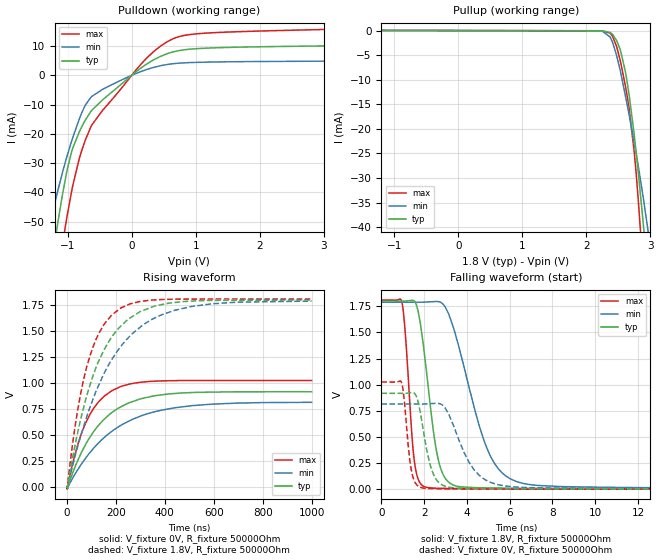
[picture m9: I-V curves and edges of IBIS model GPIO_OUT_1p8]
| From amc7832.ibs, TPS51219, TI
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|   Model
[Model]   GPIO_OUT_1p8
Model_type   Output
Polarity   Non-Inverting
Vmeas = 0.9
Vref = 1.8
Cref = 1pF
Rref = 1000000
|   typ   min   max
C_comp   1pF   1pF   1pF
[Voltage Range]   1.8   1.79   1.81
[Temperature Range]   27   125   -40
[Pullup Reference]   1.8   1.79   1.81
[Pulldown Reference]   -0   -0   -0
[Power Clamp Reference]   1.8   1.79   1.81
[GND Clamp Reference]   -0   -0   -0
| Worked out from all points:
|   slope of the pulldown table from 0 to 0.27 V, typ, clamps not added: 62.1 ohm
|   slope of the pullup table from 0 to 0.27 V, typ, clamps not added: 48 kohm
|   falling waveform, V_fixture 1.8V, R_fixture 50000Ohm: 20-80 % time 660ps typ, 1.47ns min, 358ps max; typ from 1.8 V to 0.004 V
|   rising waveform, V_fixture 0V, R_fixture 50000Ohm: 20-80 % time 163ns typ, 226ns min, 109ns max; typ from 0.002 V to 0.918 V
|   rising waveform, V_fixture 1.8V, R_fixture 50000Ohm: 20-80 % time 152ns typ, 208ns min, 104ns max; typ from 0.004 V to 1.8 V
|   falling waveform, V_fixture 0V, R_fixture 50000Ohm: 20-80 % time 532ps typ, 1.15ns min, 296ps max; typ from 0.918 V to 0.002 V
[Pulldown]
|   Voltage   I(typ)   I(min)   I(max)
-1.8V     -153.5mA   -105.7mA   -209mA
-1.309V   -73.18mA   -53.88mA   -99.6mA
-1.168V   -52.55mA   -40.82mA   -71.78mA
-1.082V   -41.03mA   -33.39mA   -58mA
-1.017V   -33.45mA   -28.23mA   -49.31mA
-919.8mV  -24.93mA   -21.36mA   -37.74mA
-784.8mV  -17.87mA   -13.12mA   -26.12mA
-622.8mV  -11.97mA   -7.251mA   -17.02mA
154.8mV   2.634mA    1.352mA    4.008mA
559.8mV   7.408mA    3.695mA    11.5mA
1.138V    9.23mA     4.469mA    14.36mA
3.595V    10.18mA    4.865mA    15.94mA
[Pullup]
|   Voltage   I(typ)   I(min)   I(max)
-1.8V     37.49uA    30.22uA    47.14uA
2.147V    -45.6uA    -47.64uA   -56.55uA
2.369V    -385.3uA   -1.286mA   -520.2uA
2.471V    -2.035mA   -5.037mA   -3.243mA
2.52V     -3.597mA   -7.642mA   -5.638mA
2.628V    -9.791mA   -14.5mA    -12.64mA
2.741V    -20.59mA   -22.4mA    -24.04mA
2.812V    -29.09mA   -27.69mA   -34.73mA
2.882V    -38.44mA   -33.47mA   -47.71mA
2.893V    -39.94mA   -34.39mA   -49.83mA
3.038V    -61.2mA    -47.6mA    -80.07mA
3.595V    -152.1mA   -106mA     -204.8mA
[Ramp]
R_load = 50000
|   typ   min   max
dV/dt_r   0.54985/1.6255e-07   0.488051/2.25521e-07   0.614753/1.08572e-07
dV/dt_f   1.07777/6.6e-10   1.06994/1.46783e-09   1.08424/3.57833e-10
[Falling Waveform]
V_fixture = 1.8V
V_fixture_min = 1.79V
V_fixture_max = 1.81V
R_fixture = 50000Ohm
C_fixture = 0F
|   Time   V(typ)   V(min)   V(max)
0s        1.8V       1.79V      1.81V
984.2ps   1.8V       1.79V      1.768V
1.466ns   1.808V     1.79V      423mV
1.73ns    1.693V     1.79V      92.9mV
2.711ns   243.4mV    1.794V     9.714mV
3.805ns   22.78mV    1.219V     6.281mV
4.99ns    14.15mV    366.8mV    5.045mV
6.018ns   11.18mV    101.9mV    4.367mV
14.03ns   4.765mV    13.88mV    3.009mV
1us       3.902mV    6.729mV    2.919mV
[Rising Waveform]
V_fixture = 0V
V_fixture_min = 0V
V_fixture_max = 0V
R_fixture = 50000Ohm
C_fixture = 0F
|   Time   V(typ)   V(min)   V(max)
0s        1.97mV     3.048mV    1.633mV
779ps     -5.04mV    3.14mV     -19.51mV
21.43ns   125.8mV    78.91mV    211.5mV
44.24ns   258mV      169mV      411mV
90.52ns   469.1mV    323.6mV    685.4mV
152.9ns   655.1mV    479.3mV    877mV
221.2ns   774mV      596.6mV    969.7mV
357.2ns   879.3mV    724.6mV    1.019V
511.7ns   910.4mV    784.3mV    1.026V
1us       918.4mV    816.5mV    1.026V
[Rising Waveform]
V_fixture = 1.8V
V_fixture_min = 1.79V
V_fixture_max = 1.81V
R_fixture = 50000Ohm
C_fixture = 0F
|   Time   V(typ)   V(min)   V(max)
0s        3.902mV    6.729mV    2.919mV
40.98ns   495.8mV    368.3mV    703.7mV
80.22ns   875.5mV    675.4mV    1.156V
132.2ns   1.227V     994.3mV    1.489V
183.3ns   1.446V     1.23V      1.658V
248.7ns   1.614V     1.433V     1.754V
308.5ns   1.698V     1.558V     1.79V
441.9ns   1.778V     1.703V     1.809V
593.1ns   1.797V     1.764V     1.81V
1us       1.8V       1.79V      1.81V
[Falling Waveform]
|Gnd
V_fixture = 0V
V_fixture_min = 0V
V_fixture_max = 0V
R_fixture = 50000Ohm
C_fixture = 0F
|   Time   V(typ)   V(min)   V(max)
0s        918.4mV    816.3mV    1.026V
940.5ps   918mV      816.2mV    1.025V
1.375ns   924.2mV    816.1mV    215.9mV
1.643ns   886.5mV    816.1mV    46.17mV
2.451ns   136.2mV    821.3mV    6.191mV
2.978ns   30.11mV    780.2mV    5.032mV
3.805ns   10.35mV    383.7mV    3.659mV
5.812ns   6.223mV    31.88mV    2.594mV
17.48ns   2.294mV    5.1mV      1.631mV
1us       1.97mV     3.048mV    1.633mV
